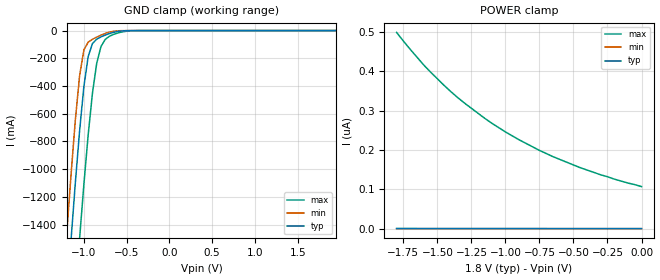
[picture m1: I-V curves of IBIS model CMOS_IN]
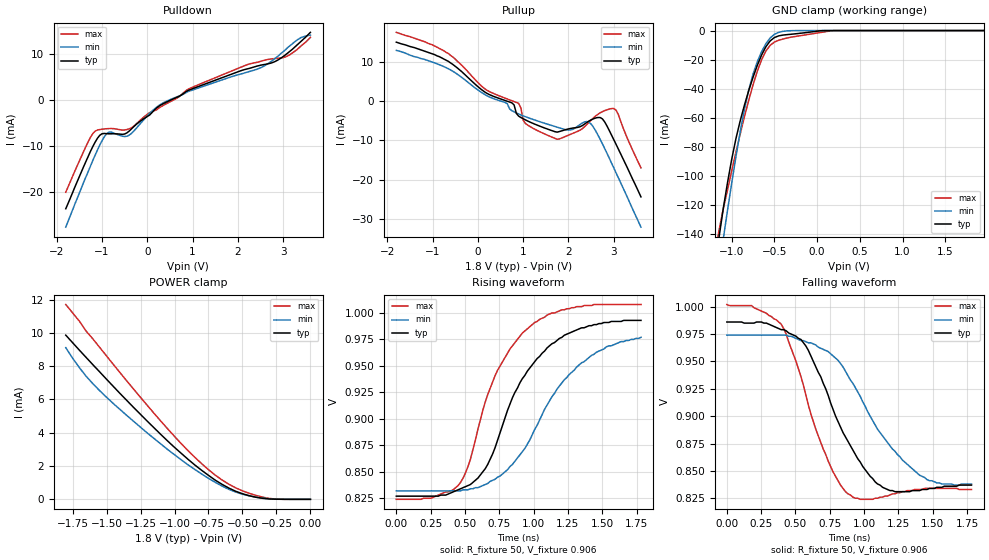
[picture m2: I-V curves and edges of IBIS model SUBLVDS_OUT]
| Texas Instruments Incorporated
| SN65LVDS315: CAMERA PARALLEL RGB TO MIPI CSI-1 SERIAL CONVERTER
| Marketing part#   Voltage Range   Package-type   #pins/pkg drawing
| SN65LVDS315RGE   1.8v - 1.95v   QFN   24-pin RGE
[IBIS Ver]   4.0
[File Name]   sn65lvds315.ibs
[File Rev]   1.0
[Date]   01/11/2011
[Source]   Texas Instruments Incorporated.
   Analog-eLab, HPA
   12500 TI Blvd
   Dallas, TX -75243
   For Support e-mail: elab_scm_ibis@list.ti.com
[Notes]   Revision History
   Rev 1.0: 01/11/2011
   - Spin model built from SN65LVDS301 v1.0
   - warnings related to IV-VT mismatch are as per lvds301 1.0 model
[Disclaimer] This model is designed as an aid for customers of Texas Instruments.
 TI and its licensors and suppliers make no warranties, either expressed
 or implied, with respect to this  model, including the warranties of
 merchantability or fitness for a particular purpose.
 The model is provided solely on an "as is" basis. The entire risk as to
 its quality and performance is with the customer.
[Copyright] (C)Copyright 2011 Texas Instruments Incorporated.
   All rights reserved.
[Component]   SN65LVDS315RGE
[Manufacturer]  Texas Instruments Incorporated
[Package]   |24-pin QFN 0.5mm Pitch
|   typ   min   max
R_pkg   0.201   0.173   0.227
L_pkg   1.401n   1.187n   1.597n
C_pkg   0.176p   0.169p   0.185p
[Pin] signal_name  model_name   R_pin   L_pin   C_pin
   1   GNDD   GND   0.21406  1.50931nH  0.16680pF
   2   DOUTN   SUBLVDS_OUT   0.20284  1.41905nH  0.17981pF
   3   DOUTP   SUBLVDS_OUT   0.19481  1.35813nH  0.17449pF
   4   CLKN   SUBLVDS_OUT   0.19484  1.35834nH  0.17494pF
   5   CLKP   SUBLVDS_OUT   0.20227  1.41485nH  0.18522pF
   6   GNDA   GND   0.11262  1.23659nH  0.21213pF
   7   TXEN   CMOS_IN   0.20836  1.46541nH  0.16918pF
   8   MODE   CMOS_IN   0.18258  1.26495nH  0.17603pF
   9   VDDA   POWER   0.08816  0.90019nH  0.19763pF
   10   D0   CMOS_IN   0.19446  1.35154nH  0.17499pF
   11   D1   CMOS_IN   0.19942  1.38795nH  0.18195pF
   12   D2   CMOS_IN   0.21992  1.54721nH  0.17450pF
   13   D3   CMOS_IN   0.22661  1.59691nH  0.17393pF
   14   D4   CMOS_IN   0.21025  1.46675nH  0.18417pF
   15   D5   CMOS_IN   0.19595  1.35784nH  0.17541pF
   16   DCLK   CMOS_IN   0.19546  1.35413nH  0.17671pF
   17   GNDD   GND   0.10094  1.04940nH  0.22249pF
   18   D6   CMOS_IN   0.21377  1.49921nH  0.17309pF
   19   D7   CMOS_IN   0.20836  1.45921nH  0.16940pF
   20   VS   CMOS_IN   0.18230  1.25915nH  0.17428pF
   21   HS   CMOS_IN   0.17248  1.18734nH  0.16972pF
   22   VDDIO   POWER   0.09215  0.94554nH  0.20674pF
   23   VDDD   POWER   0.09584  0.99831nH  0.21038pF
   24   FSEL   CMOS_IN   0.20998  1.47760nH  0.17025pF
[Diff_pin]   inv_pin   vdiff   tdelay_typ   tdelay_min   tdelay_max
   3   2   0.00   0   0   0
   5   4   0.00   0   0   0
| Models and submodels in the file (2): CMOS_IN (Input), SUBLVDS_OUT (3-state)
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|   CMOS_IN Model
[Model]   CMOS_IN
Model_type   Input
Vinh = 1.26   |0.7VDD
Vinl = 0.24   |0.3VDD
|   typ   min   max
C_comp   1.95pF   1.90pF   2.00pF
|   typ   min   max
[Temperature Range]   25.0   85   -40
[Voltage range]   1.8V   1.65V   1.95V
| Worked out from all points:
|   GND clamp passes 1 mA (typ) near -0.50 V on its own axis
[GND Clamp]
|Voltage   I(typ)   I(min)   I(max)
-1.8V     -7.58A     -7.13A     -8.39A
-1.2V     -1.95A     -1.46A     -2.78A
-1.15V    -1.51A     -1.04A     -2.34A
-1.1V     -1.1A      -646mA     -1.91A
-1.05V    -723mA     -325mA     -1.5A
-1V       -404mA     -140mA     -1.11A
-950mV    -188mA     -83.5mA    -754mA
-900mV    -94.1mA    -62.8mA    -453mA
-850mV    -62.2mA    -47mA      -236mA
-800mV    -45.5mA    -32.9mA    -115mA
-600mV    -6.07mA    -1.65mA    -16.8mA
1.95V     146pA      16.7pA     107nA
[Power_clamp]
| Note that the[POWER_clamp]voltage table is referenced to Vcc
| and is calculated using Vtable=Vcc - Vmeasured.
|Voltage   I(typ)   I(min)   I(max)
-1.8V     473pA      30pA       499nA
-1.7V     439pA      29.1pA     456nA
-1.6V     407pA      28.2pA     416nA
-1.4V     352pA      26.4pA     348nA
-1.3V     328pA      25.5pA     319nA
-1.15V    295pA      24.2pA     280nA
-1V       265pA      22.9pA     246nA
-750mV    223pA      20.6pA     199nA
-650mV    208pA      19.8pA     183nA
-450mV    181pA      18pA       155nA
-200mV    152pA      15.8pA     126nA
0V        130pA      12.8pA     107nA
|   SUBLVDS_OUT Model
[Model]   SUBLVDS_OUT
Model_type   3-state
Vmeas = 0.9   |Reference voltage for timing measurements
Cref = 1pF   |Timing specification test load capacitance value
Rref = 50
| variable   typ   min   max
C_comp   2.25pF   2.08pF   2.37pF
|   typ   min   max
[Temperature Range]   25.0   85   -40
[Voltage range]   1.8V   1.65V   1.95V
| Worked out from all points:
|   slope of the pulldown table from 0 to 0.27 V, typ, clamps not added: 117 ohm
|   slope of the pullup table from 0 to 0.27 V, typ, clamps not added: 128 ohm
|   GND clamp passes 1 mA (typ) near -0.08 V on its own axis
|   POWER clamp passes 1 mA (typ) near -0.67 V on its own axis
|   rising waveform, R_fixture 50, V_fixture 0.906: 20-80 % time 371ps typ, 438ps min, 322ps max; typ from 0.827 V to 0.993 V
|   falling waveform, R_fixture 50, V_fixture 0.906: 20-80 % time 320ps typ, 406ps min, 264ps max; typ from 0.986 V to 0.837 V
[Pulldown]
|Voltage   I(typ)   I(min)   I(max)
-1.8V     -23.7mA    -27.7mA    -20.1mA
-1.2V     -10.1mA    -13.1mA    -7.3mA
-1.05V    -7.72mA    -9.85mA    -6.46mA
-900mV    -7.36mA    -7.4mA     -6.28mA
-400mV    -6.79mA    -7.68mA    -6.31mA
350mV     -837uA     -650uA     -1.22mA
1.15V     2.99mA     2.66mA     3.39mA
2.45V     7.42mA     6.78mA     8.24mA
2.8V      8.26mA     8.87mA     8.98mA
3.1V      10.2mA     11.4mA     9.57mA
3.4V      12.8mA     13.6mA     11.8mA
3.6V      14.7mA     14.1mA     13.6mA
[Pullup]
|   Voltage   I(typ)   I(min)   I(max)
| Note that the[Pullup]voltage table is referenced to Vcc
| and is calculated using Vtable=Vcc - Vmeasured.
-1.8V     15mA       12.9mA     17.5mA
-650mV    10.1mA     8.22mA     12.1mA
150mV     2.33mA     1.69mA     3.15mA
750mV     -447uA     -2.45mA    82.7uA
900mV     -3.83mA    -3.28mA    -572uA
1.05V     -4.8mA     -3.98mA    -5.71mA
1.45V     -6.76mA    -5.57mA    -8.25mA
1.8V      -7.76mA    -6.82mA    -9.64mA
2.45V     -5.1mA     -5.35mA    -5.44mA
2.75V     -4.55mA    -10.9mA    -2.69mA
3.05V     -11mA      -18.3mA    -2.31mA
3.6V      -24.4mA    -32.1mA    -17mA
[GND Clamp]
|Voltage   I(typ)   I(min)   I(max)
-1.95V    -492mA     -507mA     -485mA
-1.15V    -143mA     -164mA     -138mA
-1.1V     -123mA     -144mA     -123mA
-1.05V    -105mA     -124mA     -110mA
-950mV    -74.2mA    -86.6mA    -83.6mA
-850mV    -51.1mA    -54mA      -59.1mA
-800mV    -41.2mA    -40.7mA    -47.8mA
-750mV    -32.1mA    -29.9mA    -37.3mA
-650mV    -16.8mA    -14.5mA    -20.1mA
-500mV    -4.79mA    -2.58mA    -7.91mA
200mV     -1.73nA    -14.2nA    -1.19nA
1.95V     308nA      31.1uA     1.06nA
[POWER Clamp]
|Voltage   I(typ)   I(min)   I(max)
-1.8V     9.86mA     9.11mA     11.7mA
-1.7V     8.96mA     7.91mA     10.7mA
-1.65V    8.52mA     7.39mA     10.1mA
-1.45V    6.78mA     5.75mA     8.1mA
-1.2V     4.69mA     3.98mA     5.64mA
-1V       3.12mA     2.68mA     3.78mA
-850mV    2.06mA     1.79mA     2.52mA
-700mV    1.15mA     1.02mA     1.45mA
-550mV    485uA      438uA      690uA
-350mV    58uA       68.5uA     128uA
-250mV    5.84uA     12uA       13.3uA
0V        3.03nA     42.8nA     1.06nA
[Ramp]
|   typ   min   max
dV/dt_r   0.095V/332.8ps  0.085V/425.4ps  0.106V/289.9ps
dV/dt_f   0.096V/354.2ps  0.086V/443.5ps  0.107V/282.7ps
R_load = 50ohm  | Note: The measurement is single-ended with 50ohm
|   to common mode voltage.
[Rising Waveform]
R_fixture = 50
V_fixture = 0.906
V_fixture_min = 0.903
V_fixture_max = 0.913
|Time   V(typ)   V(min)   V(max)
0s        827mV      832mV      824mV
450ps     833mV      832mV      837mV
522ps     837mV      833mV      855mV
594ps     844mV      835mV      890mV
738ps     880mV      845mV      946mV
864ps     925mV      860mV      972mV
1.008ns   954mV      890mV      991mV
1.17ns    974mV      928mV      1.001V
1.314ns   984mV      949mV      1.006V
1.782ns   993mV      977mV      1.008V
[Falling Waveform]
R_fixture = 50
V_fixture = 0.906
V_fixture_min = 0.903
V_fixture_max = 0.913
|Time   V(typ)   V(min)   V(max)
0s        986mV      974mV      1.002V
180ps     985mV      974mV      1.001V
396ps     979mV      974mV      984mV
504ps     973mV      971mV      950mV
576ps     964mV      968mV      919mV
738ps     919mV      959mV      859mV
882ps     877mV      937mV      829mV
1.098ns   838mV      888mV      825mV
1.404ns   832mV      846mV      833mV
1.782ns   837mV      838mV      833mV
